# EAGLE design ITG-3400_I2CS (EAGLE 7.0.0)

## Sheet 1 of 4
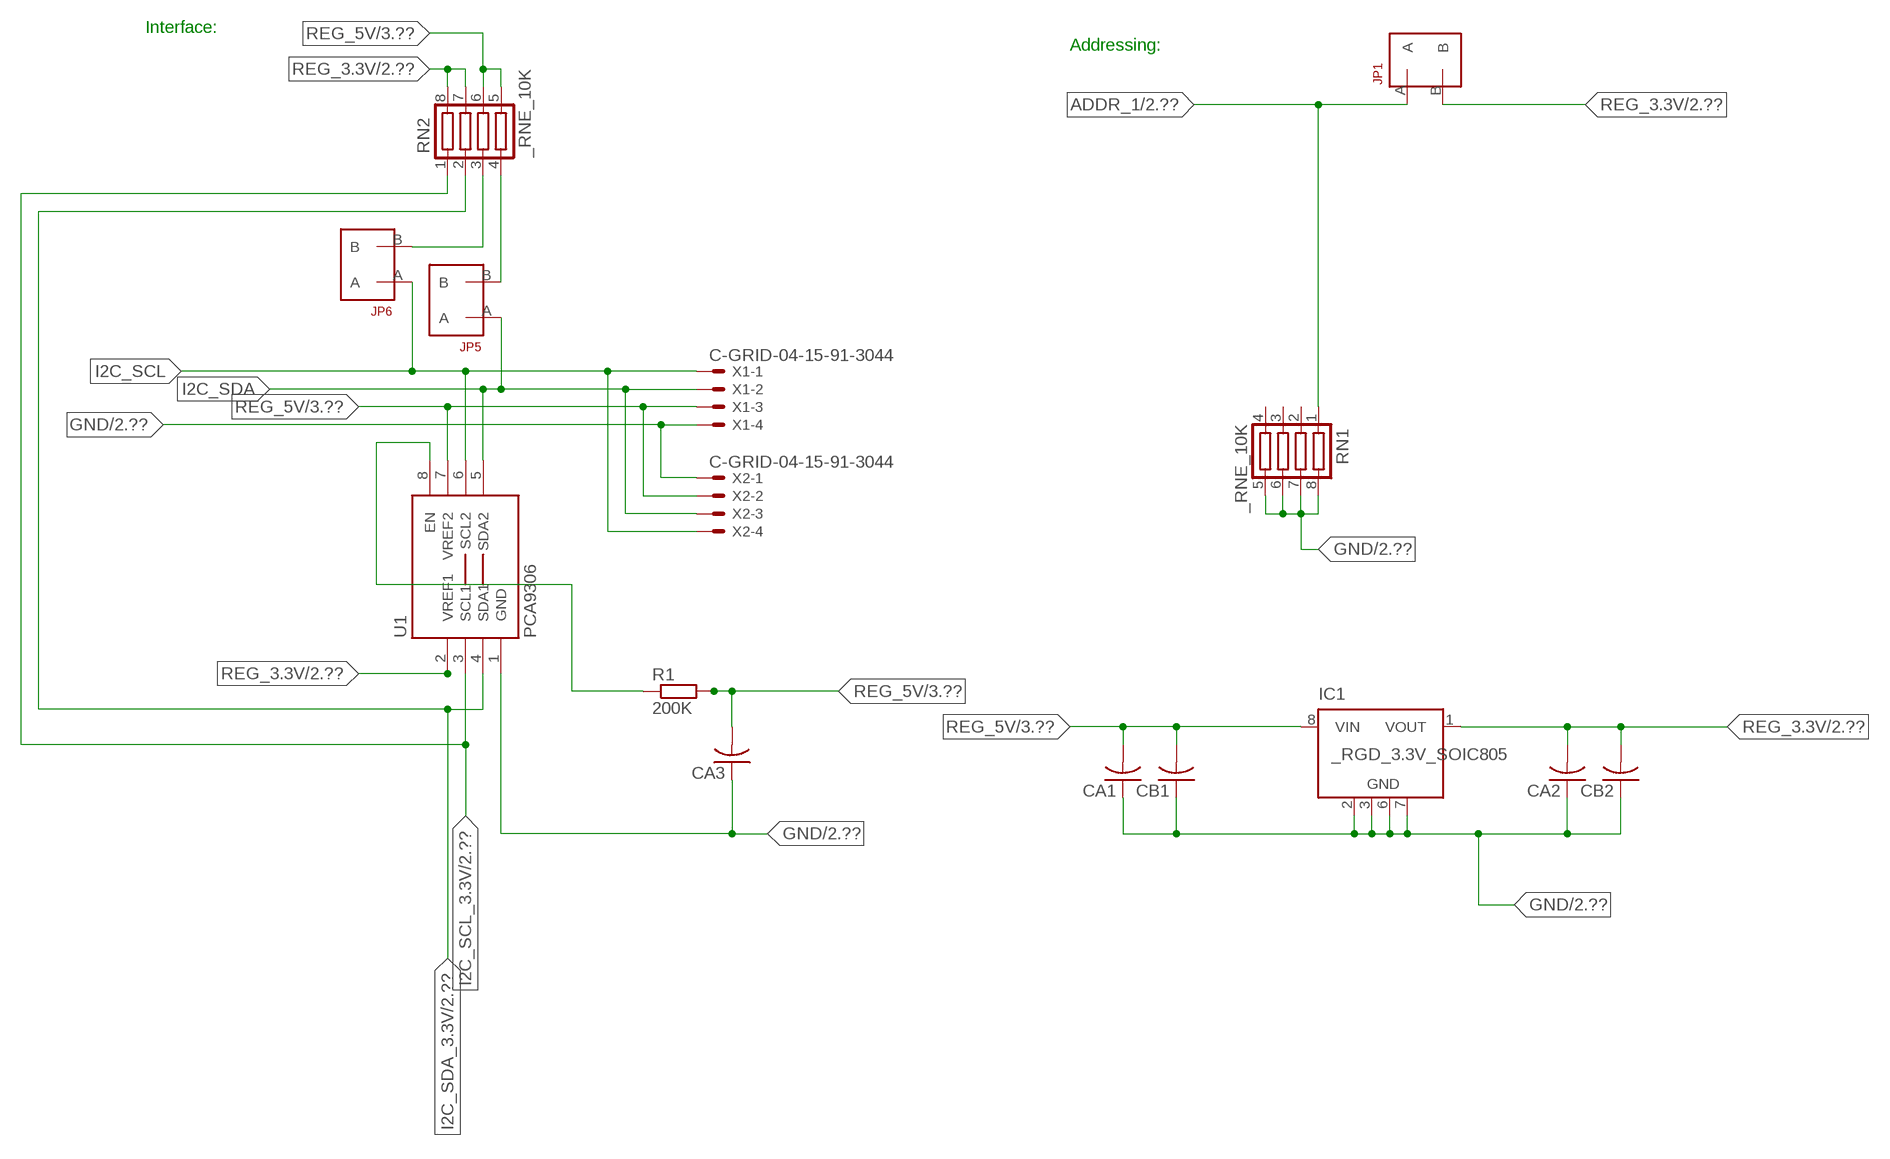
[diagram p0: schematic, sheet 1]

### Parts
CA1  CC1206KRX7R9BB104  [.1UF]
CA2  CC1206KRX7R9BB104  [.1UF]
CA3  CC1206KRX7R9BB104  [.1UF]
CB1  TMK316F106ZL-TC1206K  [TMK316F106ZL-T]
CB2  TMK316F106ZL-TC1206K  [TMK316F106ZL-T]
IC1  _RGD_3.3V_SOIC805  [_RGC_3.3V_SOIC8]
JP1  JUMPER_1X2_2MM  [JUMPER_1X2_2MM]
JP5  JUMPER_1X2_2MM  [JUMPER_1X2_2MM]
JP6  JUMPER_1X2_2MM  [JUMPER_1X2_2MM]
R1  200K  RESISTOR_SMT-0603  [R603]
RN1  _RNE_10K  [RNE]
RN2  _RNE_10K  [RNE]
U1  PCA9306  PCA9306_NCD  [PSOP-8]
X1  C-GRID-04-15-91-3044  [15-91-04]
X2  C-GRID-04-15-91-3044  [15-91-04]

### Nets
ADDR_1: JP1.A RN1.1 ; also sheet 2
GND: CA1.1 CA2.1 CA3.1 CB1.1 CB2.1 IC1.2(GND) IC1.3(GND) IC1.6(GND) IC1.7(GND) RN1.5 RN1.6 RN1.7 RN1.8 U1.1(GND) X1.4 X2.1 ; also sheet 2,3
I2C_SCL: JP6.A U1.6(SCL2) X1.1 X2.4
I2C_SCL_3.3V: RN2.1 U1.3(SCL1) ; also sheet 2
I2C_SDA: JP5.A U1.5(SDA2) X1.2 X2.3
I2C_SDA_3.3V: RN2.2 U1.4(SDA1) ; also sheet 2
N$1: JP6.B RN2.3
N$2: JP5.B RN2.4
N$3: R1.1 U1.8(EN)
REG_3.3V: CA2.2 CB2.2 IC1.1(VOUT) JP1.B RN2.7 RN2.8 U1.2(VREF1) ; also sheet 2
REG_5V: CA1.2 CA3.2 CB1.2 IC1.8(VIN) R1.2 RN2.5 RN2.6 U1.7(VREF2) X1.3 X2.2 ; also sheet 3
Unconnected: IC1.4(NC) IC1.5(NC) RN1.2 RN1.3 RN1.4

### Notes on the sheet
- Interface:
- Addressing:

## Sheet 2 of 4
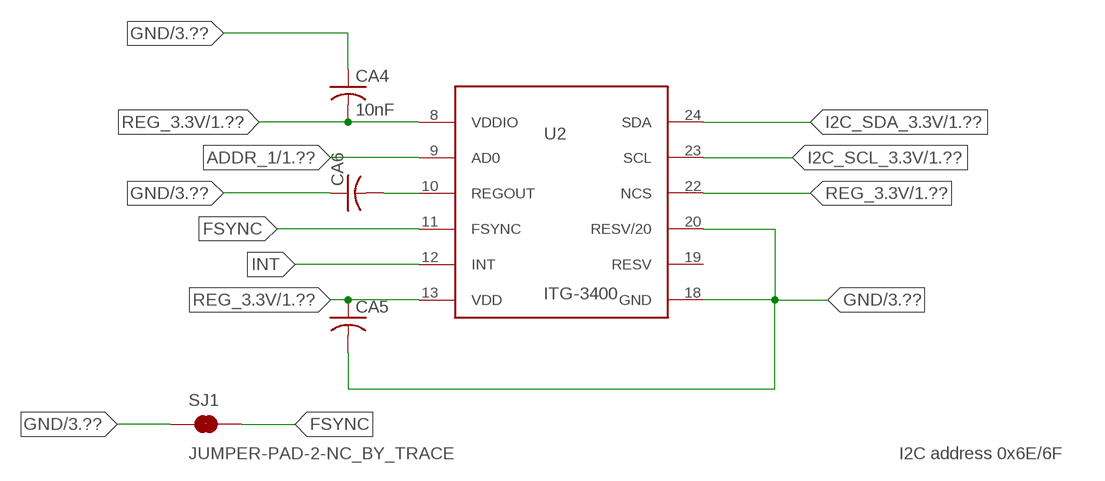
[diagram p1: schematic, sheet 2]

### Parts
CA4  10nF  CC1206KRX7R9BB104  [.1UF]
CA5  CC1206KRX7R9BB104  [.1UF]
CA6  CC1206KRX7R9BB104  [.1UF]
SJ1  JUMPER-PAD-2-NC_BY_TRACE  [PAD-JUMPER-2-NC_BY_TRACE_YES_SILK]
U2  ITG-3400  [QFN-24]

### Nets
ADDR_1: U2.9(AD0) ; also sheet 1
FSYNC: SJ1.2 U2.11(FSYNC)
GND: CA4.1 CA5.2 CA6.1 SJ1.1 U2.18(GND) U2.20(RESV/20) ; also sheet 1,3
I2C_SCL_3.3V: U2.23(SCL) ; also sheet 1
I2C_SDA_3.3V: U2.24(SDA) ; also sheet 1
INT: U2.12(INT)
N$4: CA6.2 U2.10(REGOUT)
REG_3.3V: CA4.2 CA5.1 U2.8(VDDIO) U2.13(VDD) U2.22(NCS) ; also sheet 1
Unconnected: U2.19(RESV)

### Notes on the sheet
- I2C address 0x6E/6F

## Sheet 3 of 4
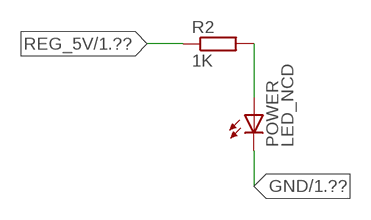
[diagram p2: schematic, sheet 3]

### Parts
POWER  LED_NCD  [CHIPLED_0603]
R2  1K  RESISTOR_SMT-0402  [R402]

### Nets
GND: POWER.C ; also sheet 1,2
N$5: POWER.A R2.2
REG_5V: R2.1 ; also sheet 1

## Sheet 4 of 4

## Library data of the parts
CA1-CA6 = NCD_ULTIMATE_LIBRARY:CC1206KRX7R9BB104: Capacitor CA .1uF 50V SMT C1206K CC1206KRX7R9BB104
CB1 CB2 = NCD_ULTIMATE_LIBRARY:TMK316F106ZL-T: Capacitor CB 10uF SMT 1206 TMK316F106ZL-T
IC1 = NCD_ULTIMATE_LIBRARY:_RGD_3.3V_SOIC8: Regulator Linear 3.3V Chip Positive VOLTAGE REGULATOR Digikey 497-1199-2-ND/L78L33ACD13TR
JP1 JP5 JP6 = NCD_ULTIMATE_CONNECTORS:JUMPER_1X2_2MM
POWER = NCD_ULTIMATE_LIBRARY:LED_NCD: LED Digikey 754-1132-2-ND/APT2012SRCPRV
R1 R2 = NCD_ULTIMATE_LIBRARY:RESISTOR_SMT: NCD Resistor
RN1 RN2 = NCD_ULTIMATE_LIBRARY:_RNE_10K: Resistor Array RNE SMT 10K x 4 Single Resistor Source: http://www.ctscorp.com/components/Datasheets/CTSChipArrayDs.pdf Digikey 742C083103JPTR-ND/742C083103JP; OC_FARNELL: unknown; OC_NEWARK: unknown
SJ1 = NCD_ULTIMATE_CONNECTORS:JUMPER-PAD-2-NC_BY_TRACE
U1 = NCD_ULTIMATE_LIBRARY:PCA9306_NCD: NCD Bidirectional I2C level shifter. NOT compatible with all available part number pinout schemes- DOUBLE CHECK!!!; PROD_ID: IC-10023
U2 = NCD_ULTIMATE_bhaskar:ITG-3400
X1 X2 = NCD_ULTIMATE_CONNECTORS:C-GRID-04: CONNECTOR 4-Pos I2C wire to board 2.54 mm (0.100") pitch header Digikey WM1342-ND/0015912045; OC_FARNELL: unknown; OC_NEWARK: unknown

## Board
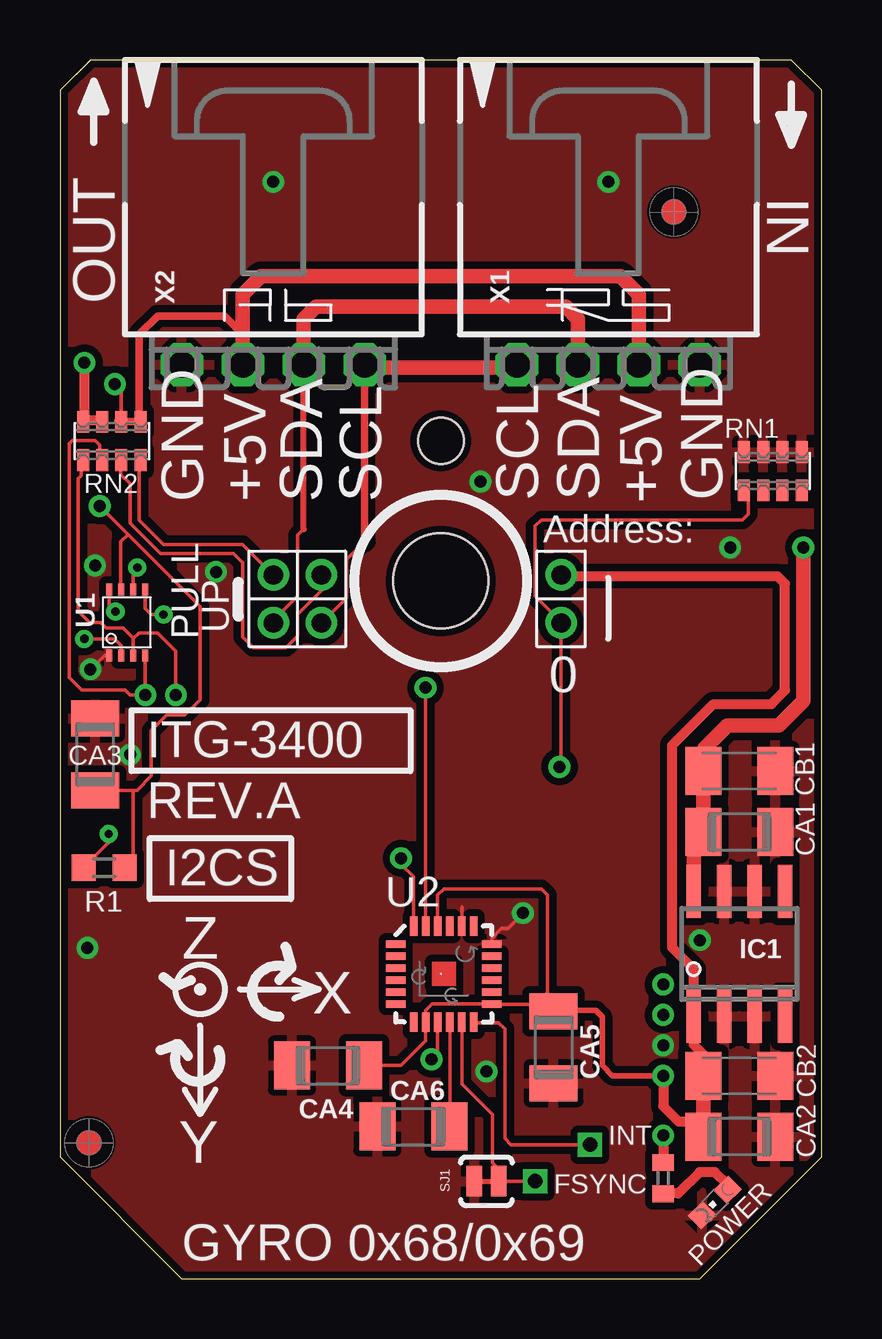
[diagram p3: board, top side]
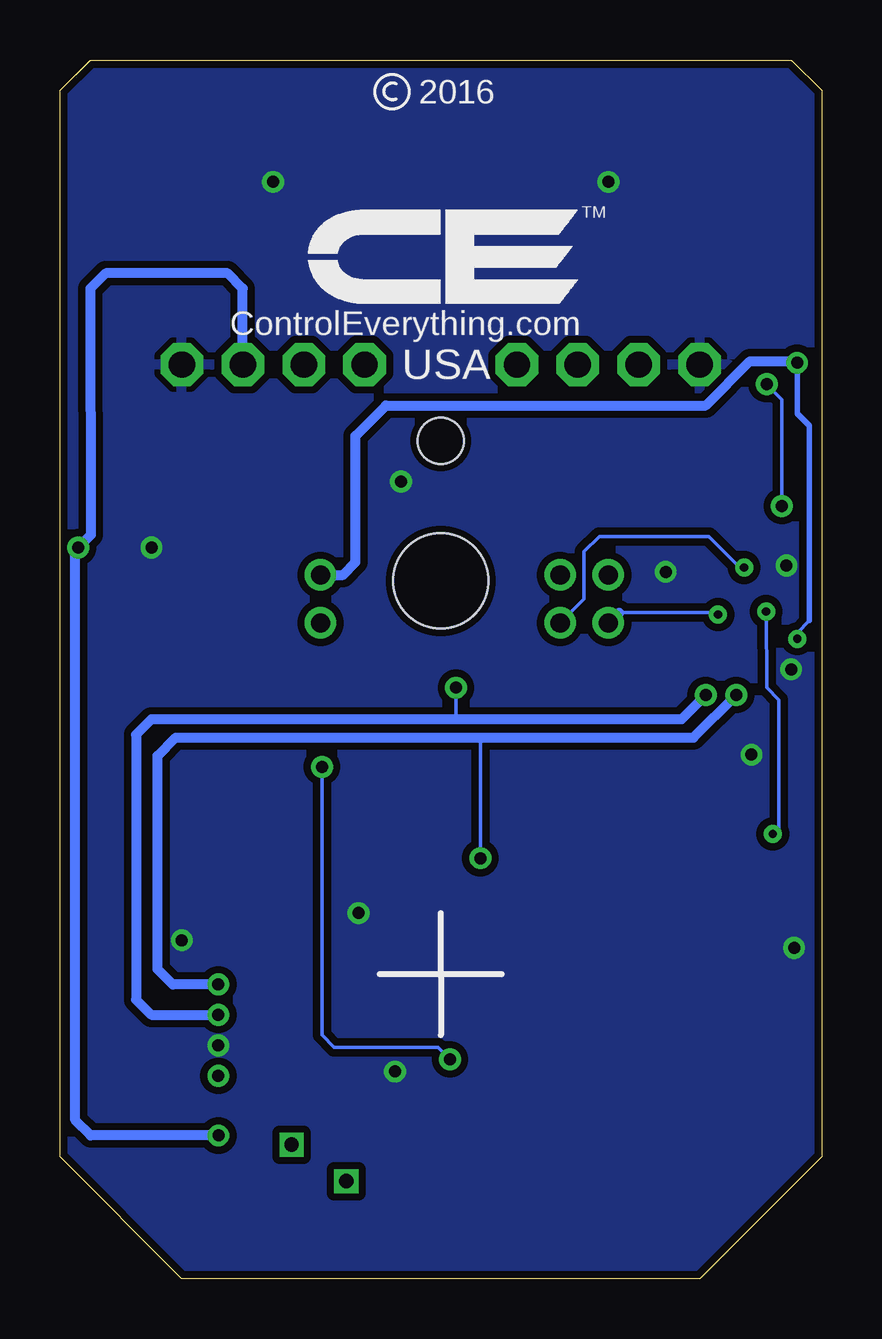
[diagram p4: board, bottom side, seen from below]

Size 31.75 x 50.8 mm. Coordinates in mm from the lower left corner, seen from the top.
Outline: 48 segments
Copper layers (1*16): Top 0.035mm / dielectric 1.5mm / Bottom 0.035mm
Design rules "default": minimum track width 5mil, minimum drill 24mil, track to track 5mil, track to pad 5mil, pad to pad 5mil, via to via 5mil, smd to smd 5mil, copper to edge 10mil, drill to drill 8mil, minimum pad ring 10mil, minimum via ring 8mil, stop-mask expansion 2mil, vias tented up to drill 0mil, thermal gap 10mil
Holes 3.96 mm at 15.88,29.08
Holes 1.91 mm at 15.88,34.93

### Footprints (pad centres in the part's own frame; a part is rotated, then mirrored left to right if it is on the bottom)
.1UF = smd 1.5 x 2: 1 -1.5,0; 2 1.5,0
TMK316F106ZL-T = smd 1.5 x 2: 1 -1.5,0; 2 1.5,0
_RGC_3.3V_SOIC8 = smd 0.6 x 2.2: 1 -1.905,-2.6; 2 -0.635,-2.6; 3 0.635,-2.6; 4 1.905,-2.6; 5 1.905,2.6; 6 0.635,2.6; 7 -0.635,2.6; 8 -1.905,2.6
JUMPER_1X2_2MM = drill 0.8: A 0,2; B 0,0
CHIPLED_0603 = smd 0.8 x 0.876: A 0,-0.75; C 0,0.75
R603 = smd 1 x 1.1: 1 -0.85,0; 2 0.85,0
R402 = smd 0.7 x 0.9: 1 -0.65,0; 2 0.65,0
RNE = smd 0.5 x 0.9: 1 -1.2,-0.8; 2 -0.4,-0.8; 3 0.4,-0.8; 4 1.2,-0.8; 5 1.2,0.8; 6 0.4,0.8; 7 -0.4,0.8; 8 -1.2,0.8
PAD-JUMPER-2-NC_BY_TRACE_YES_SILK = smd 0.635 x 1.27: 1 -0.508,0; 2 0.508,0
PSOP-8 = smd 0.25 x 0.5: 1 -0.73,-1.37; 2 -0.23,-1.37; 3 0.27,-1.37; 4 0.77,-1.37; 5 0.77,1.38; 6 0.27,1.38; 7 -0.23,1.38; 8 -0.73,1.38
QFN-24 = smd 0.8 x 0.3: 1 -2,1.25; 2 -2,0.75; 3 -2,0.25; 4 -2,-0.25; 5 -2,-0.75; 6 -2,-1.25; 13 2,-1.25; 14 2,-0.75; 15 2,-0.25; 16 2,0.25; 17 2,0.75; 18 2,1.25 | smd 0.3 x 0.8: 7 -1.25,-2; 8 -0.75,-2; 9 -0.25,-2; 10 0.25,-2; 11 0.75,-2; 12 1.25,-2; 19 1.25,2; 20 0.75,2; 21 0.25,2; 22 -0.25,2; 23 -0.75,2; 24 -1.25,2
15-91-04 = drill 1.1 pad 1.778 octagon: 1 -3.81,-7.62; 2 -1.27,-7.62; 3 1.27,-7.62; 4 3.81,-7.62

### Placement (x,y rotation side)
CA1  28.32,18.62 180 top
CA2  28.32,5.92 180 top
CA3  1.46,21.86 270 top
CA4  11.18,8.89 0 top
CA5  20.57,9.65 270 top
CA6  14.73,6.35 0 top
CB1  28.32,21.16 180 top
CB2  28.32,8.46 180 top
IC1  28.32,13.54 0 top
JP1  20.89,29.34 180 top
JP5  8.89,29.34 180 top
JP6  10.9,29.34 180 top
POWER  27.3,3.18 135 top
R1  1.84,17.13 0 top
R2  25.15,4.19 270 top
RN1  29.72,33.66 0 top
RN2  2.16,34.93 0 top
SJ1  17.78,4.06 0 top
U1  2.79,27.36 0 top
U2  16,12.7 0 top
U$5  [VISION_REF10]  1.21,5.66 90 top
U$28  [VISION_REF10]  25.59,44.46 90 top
X1  22.86,45.72 0 top
X2  8.89,45.72 0 top

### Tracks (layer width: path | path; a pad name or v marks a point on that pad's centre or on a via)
ADDR_1  (via drill 0.5)
  Top 0.152: RN1.1 28.7,32.78 28.7,31.88 28.45,31.62 20.07,31.62 19.81,31.37 19.81,28.45 20.89,27.37 JP1.A 20.89,21.4 v20.83,21.34 | U2.9 15.75,9.4 v15.49,9.14
  Bottom 0.152: v15.49,9.14 16,9.65 20.32,9.65 20.83,10.16 v20.83,21.34
FSYNC  (via drill 0.6)
  Top 0.152: U2.11 16.76,10.69 16.76,8.13 18.03,6.86 18.03,4.83 18.29,4.57 SJ1.2 v19.81,4.06
GND  (via drill 0.5)
  Top 0.152: CA3.1 1.52,23.42 1.52,23.62 | U2.18 18,14.19 18.41,14.61 18.67,14.61 v19.3,15.24 | U2.20 16.75,15.48 16.76,15.49 | v1.27,25.4 1.86,25.99 U1.1
  other vias: 8.89,45.72 22.86,45.72 25.15,9.73 1.46,29.73 17.53,33.22 26.67,14.11 1.15,13.79 6.5,29.46 27.94,30.48 17.78,8.64 2.92,21.84
  pour Bottom (isolate 0.305): -0.64,5.08 -0.64,49.53 1.27,51.44 30.48,51.44 32.38,49.53 32.38,5.08 26.67,-0.63 5.08,-0.63
  pour Top (isolate 0.305): 4.45,-1.27 -1.27,4.45 -1.27,50.17 0.64,52.07 31.11,52.07 33.02,50.17 33.02,4.45 27.3,-1.27
I2C_SCL  (via drill 0.35)
  Top 0.152: 12.7,30.73 11.94,29.97 11.94,28.38 JP6.A | v3.23,29.64 3.06,29.48 U1.6
  Top 0.305: 12.7,30.73 X2.4
  Top 0.406: X2.4 12.7,37.97 | 19.05,37.97 X1.1
  Top 0.61: 12.7,37.97 19.05,37.97
  Bottom 0.152: JP6.A 9.91,28.33 9.91,30.3 9.27,30.94 4.7,30.94 3.48,29.72 v3.23,29.64
I2C_SCL_3.3V  (via drill 0.5)
  Top 0.152: RN2.1 0.89,34.07 0.89,33.48 0.77,33.35 0.77,27.83 1.23,27.36 1.7,27.36 1.93,27.13 2.64,27.13 3.06,26.71 3.06,26.68 | U2.23 15.24,14.71 v15.24,24.64 | v4.83,24.33 v4.83,24.34 4.83,26.16 4.06,26.92 3.3,26.92 3.06,26.68 | 3.06,26.68 U1.3
  Bottom 0.152: v15.24,24.64 15.24,23.32
  Bottom 0.406: v4.83,24.33 5.84,23.32 15.24,23.32 27.94,23.32 28.58,22.68 28.58,11.63 27.94,11 v25.15,11
I2C_SDA  (via drill 0.35)
  Top 0.152: JP5.A 8.89,27.44 9.91,28.45 9.91,30.99 10.16,31.24 | U1.5 3.56,27.94 3.81,27.69 v4.32,27.69
  Top 0.254: 10.16,31.24 X2.3
  Top 0.61: X2.3 10.16,40.01 10.67,40.51 21.09,40.51 21.59,40.01 X1.2
  Bottom 0.152: v4.32,27.69 4.39,27.76 8.44,27.76
  Bottom 0.406: 8.44,27.76 JP5.A
I2C_SDA_3.3V  (via drill 0.5)
  Top 0.152: RN2.2 1.65,34.14 1.65,34.75 1.46,34.94 0.51,34.94 0.38,34.81 0.38,26.37 0.38,26.36 0.38,25.07 0.91,24.54 2.72,24.54 2.92,24.33 v3.56,24.33 U1.4 | U2.24 14.73,14.72 14.73,16.76 14.22,17.27 v14.22,17.53
  Bottom 0.152: v14.22,17.53 14.22,22.56
  Bottom 0.406: v25.15,12.27 27.05,12.27 27.69,12.9 27.69,21.79 26.93,22.56 14.22,22.56 5.34,22.56 v3.56,24.33
INT  (via drill 0.6)
  Top 0.152: U2.12 17.28,10.67 18.29,10.67 18.54,10.41 18.54,5.84 18.8,5.59 v22.1,5.59
N$1
  Top 0.152: JP6.B 10.92,29.31 10.92,28.7 9.91,27.69 9.91,26.8 9.42,26.31 8.06,26.31 7.62,26.75 7.62,29.84 7.24,30.23 4.19,30.23 2.92,31.5 2.92,33.15 2.54,33.53 2.54,34.1 RN2.3
  Top 0.305: 2.54,34.02 RN2.3
N$2
  Top 0.152: JP5.B 7.62,30.61 4.32,30.61 3.3,31.62 3.3,34.07 RN2.4
  Top 0.305: 3.37,33.88 RN2.4
N$3  (via drill 0.35)
  Top 0.152: v2.31,27.81 2.06,27.91 U1.8 | R1.1 2.03,18.18 v2.03,18.54
  Bottom 0.152: v2.03,18.54 1.78,18.8 1.78,24.13 2.29,24.64 v2.31,27.81
N$4
  Top 0.152: U2.10 16.26,6.86 16.23,6.83 CA6.2
N$5
  Top 0.406: POWER.A 27.84,3.92 27.3,4.45 26.67,4.45 25.78,3.56 25.16,3.56 R2.2
REG_3.3V  (via drill 0.35, 0.5)
  Top 0.152: CA4.2 14.22,8.89 15.24,9.91 15.24,10.69 U2.8 15.24,10.71 15.24,11.18 15.51,11.45 U2.13 18.02,11.43 20.07,11.43 | 20.07,11.43 20.34,11.15 CA5.1 | U2.22 15.75,16 16,16.26 20.07,16.26 20.32,16 20.32,11.94 20.07,11.68 20.07,11.43 | v1.02,26.67 2.29,26.67 2.56,26.4 U1.2
  Top 0.229: CA5.1 20.6,11.18 22.35,11.18 22.61,10.92 22.61,8.89 23.04,8.46 v25.15,8.46
  Top 0.406: CB2.2 26.82,9.35 26.42,9.75 26.42,10.36 | v25.15,8.46 25.15,7.19 25.78,6.55 26.82,6.55 | IC1.1 26.42,12.9 25.53,13.79 25.53,22.24 27.24,23.95 29.66,23.95 30.23,24.52 30.23,28.97 29.91,29.29 20.95,29.29 JP1.B | 26.52,5.62 CA2.2 | v1.02,38.18 1.02,35.78 | 1.02,35.78 RN2.8 | 1.02,35.78 1.71,35.78 RN2.7
  Top 0.61: CB2.2 26.82,6.55 CA2.2 | 26.42,10.36 IC1.1
  Bottom 0.152: 0.51,27.43 1.02,26.92 v1.02,26.67
  Bottom 0.229: 0.51,27.43 0.51,35.56 1.02,36.07 v1.02,38.18
  Bottom 0.406: v1.02,38.18 1.08,38.24 2.99,38.24 4.83,36.4 18.16,36.4 19.43,35.13 19.43,29.87 19.94,29.34 JP1.B
REG_5V  (via drill 0.5)
  Top 0.152: RN2.6 2.56,37.01 v2.29,37.29 | R1.2 3.05,17.49 3.05,20.36 | CA3.2 3.05,20.36 | 3.05,20.36 3.21,20.36 3.81,20.96 3.81,22.86 4.45,23.5 5.21,23.5 5.84,24.13 5.84,28.02 2.83,31.03 | v1.65,32.21 2.83,31.03 | U1.7 2.54,28.76 2.54,30.73 2.83,31.03 | 2.83,31.03
  Top 0.305: 7.62,39.37 7.5,39.37 | 2.42,35.74 RN2.6 RN2.5 3.31,35.8 3.31,39.37 4.07,40.13 6.86,40.13 7.62,39.37 | X2.2 7.62,39.37
  Top 0.406: v25.15,5.97 R2.1
  Top 0.61: X2.2 7.62,41.02 8.38,41.78 23.37,41.78 24.13,41.02 X1.3 | IC1.8 26.42,18.21 CA1.2 CB1.2 26.86,21.2 26.86,22.11 27.82,23.06 29.98,23.06 30.99,24.08 v30.99,30.48
  Bottom 0.152: v1.65,32.21 1.65,36.65 v2.29,37.29
  Bottom 0.406: X1.3 24.13,41.28 24.77,41.91 29.84,41.91 30.48,41.27 30.47,31 v30.99,30.48 31.11,30.36 31.11,6.6 30.48,5.97 v25.15,5.97

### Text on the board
tPlace: GYRO 0x68/0x69
tNames: IN | OUT | GND | +5V | SDA | SCL | SCL | SDA | +5V | GND | Address: | PULL | UP | 0 | ITG-3400 | REV.A | I2CS | Z | X | INT | Y | FSYNC
bNames: 2016 | TM | ControlEverything.com | USA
